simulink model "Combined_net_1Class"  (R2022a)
settings: Solver=FixedStepAuto  StartTime=0.0  StopTime=simtime  FixedStep=1  RelTol=1e-3
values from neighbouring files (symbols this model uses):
  net = closeloop(net)    [Loadnet.m]
  SOH_predict = double(ans.SOHout(simtime))    [SimulationCycle.m]
undefined symbols (not defined in the file or in its folder): dSOC_mu_CC, dSOC_sig_CC, dv_mu_CC, dv_sig_CC, SOC_mu_CC, SOC_sig_CC, SOE_mu_CC, SOE_sig_CC, Step2_Simulink_Models, Thesis
libraries: neural x35, deeplib x1

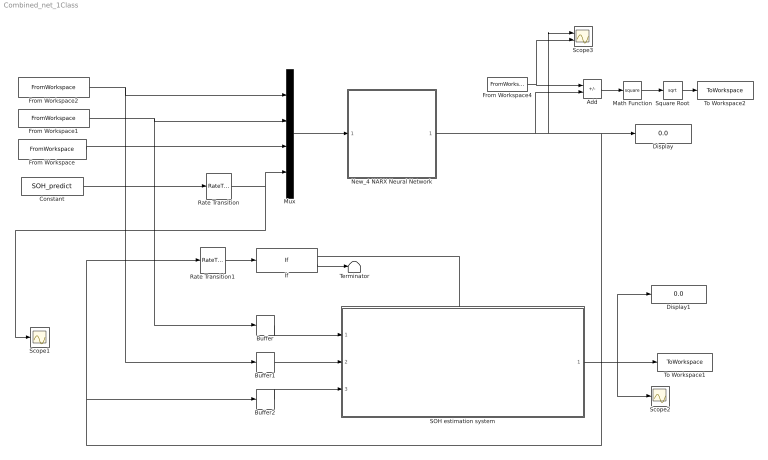
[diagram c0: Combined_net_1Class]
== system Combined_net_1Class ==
  Add : Sum  Inputs=+-
  Buffer : Buffer  N=120  OutputFrames=off
  Buffer1 : Buffer  N=120  OutputFrames=off
  Buffer2 : Buffer  N=120  OutputFrames=off
  Constant : Constant  Value=SOH_predict
  Display : Display
  Display1 : Display
  From Workspace : FromWorkspace  VariableName=Temperature
  From Workspace1 : FromWorkspace  VariableName=Voltage  SampleTime=1
  From Workspace2 : FromWorkspace  VariableName=Current  SampleTime=1
  From Workspace4 : FromWorkspace  VariableName=SOC_GT
  If : If  IfExpression=u1 < 0.6
  Math Function : Math  Operator=square
  Mux : Mux
  New_4 NARX Neural Network : Subsystem  mask{pi_input_1_delayed_1=[0;0;0;0], ai_layer_2_delayed_1=0}
      mask prompts: pi_input_1_delayed_1 "Preprocessed initial input 1 state at timestep 0."; ai_layer_2_delayed_1 "Initial layer 2 state at timestep 0."
      mask help: NARX Neural Network
  Rate Transition : RateTransition  OutPortSampleTime=1
  Rate Transition1 : RateTransition  OutPortSampleTime=1
  SOH estimation system : Subsystem
  Scope1 : Scope
  Scope2 : Scope
  Scope3 : Scope  NumInputPorts=2
  Square Root : Sqrt
  Terminator : Terminator
  To Workspace1 : ToWorkspace  VariableName=SOHout  SampleTime=-1
  To Workspace2 : ToWorkspace  VariableName=SOC_abserror  SampleTime=-1
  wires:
  Mux/1 -> New_4 NARX Neural Network/1(x)
  From Workspace/1 -> Mux/3
  Buffer/1 -> SOH estimation system/1(V)
  From Workspace1/1 -> Mux/2, Buffer/1
  If/1 -> SOH estimation system/Action
  Buffer2/1 -> SOH estimation system/3(SOC)
  Buffer1/1 -> SOH estimation system/2(I)
  Rate Transition1/1 -> If/1
  From Workspace2/1 -> Mux/1, Buffer1/1
  If/2 -> Terminator/1
  Constant/1 -> Rate Transition/1
  SOH estimation system/1(SOH) -> Scope2/1, To Workspace1/1, Display1/1
  Rate Transition/1 -> Mux/4, Scope1/1
  Math Function/1 -> Square Root/1
  Add/1 -> Math Function/1
  New_4 NARX Neural Network/1(y) -> Add/2, Scope3/1, Rate Transition1/1, Buffer2/1, Display/1
  Square Root/1 -> To Workspace2/1
  From Workspace4/1 -> Add/1, Scope3/2

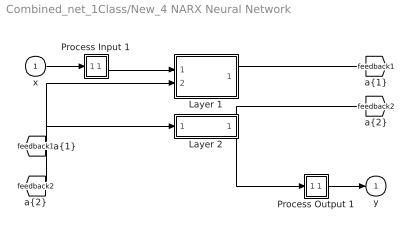
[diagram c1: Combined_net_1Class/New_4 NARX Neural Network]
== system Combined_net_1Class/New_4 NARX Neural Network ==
  x : Inport  PortDimensions=4  SampleTime=1
  Layer 1 : Subsystem
  Layer 2 : Subsystem
  Process Input 1 : Subsystem
  Process Output 1 : Subsystem
  y : Outport  InitialOutput=0
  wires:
  x/1 -> Process Input 1/1(x)
  Process Output 1/1(y) -> y/1
  Process Input 1/1(p) -> Layer 1/1("p{1}")
  Layer 1/1("a{1}") -> [feedback1]
  [feedback1] -> Layer 2/1("a{1} ")
  Layer 2/1("a{2}") -> [feedback2], Process Output 1/1(a)
  [feedback2] -> Layer 1/2("a{2} ")

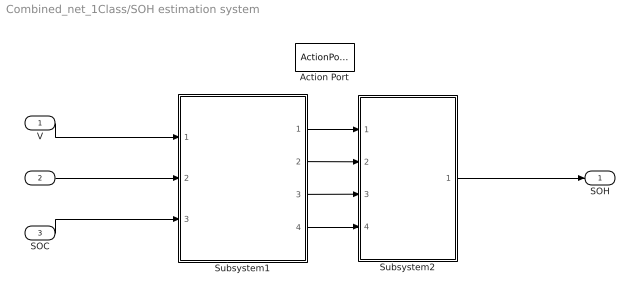
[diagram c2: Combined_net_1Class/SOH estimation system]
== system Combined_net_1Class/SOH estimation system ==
  V : Inport
  I : Inport  Port=2
  SOC : Inport  Port=3
  Action Port : ActionPort  ActionPortLabel=if(u1 < 0.6)
  Subsystem1 : Subsystem
  Subsystem2 : Subsystem
  SOH : Outport
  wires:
  Subsystem1/4(SOE) -> Subsystem2/4(SOE)
  Subsystem1/1(dSOC) -> Subsystem2/1(dSOC)
  Subsystem1/2(dv) -> Subsystem2/2(dv)
  Subsystem1/3(SOC) -> Subsystem2/3(SOC)
  Subsystem2/1(SOH) -> SOH/1
  V/1 -> Subsystem1/1(V_03)
  I/1 -> Subsystem1/2(I_03)
  SOC/1 -> Subsystem1/3(SOC_03)

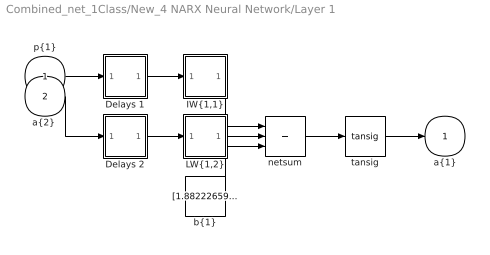
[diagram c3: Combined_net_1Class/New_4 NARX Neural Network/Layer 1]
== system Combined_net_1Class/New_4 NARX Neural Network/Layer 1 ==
  "p{1}" : Inport  PortDimensions=4  SampleTime=1
  "a{2} " : Inport  Port=2  PortDimensions=1  SampleTime=1
  Delays 1 : Subsystem
  Delays 2 : Subsystem
  "IW{1,1}" : Subsystem
  "LW{1,2}" : Subsystem
  "b{1}" : Constant  Value=[1.8822265945278056076261918860836885869503021240234375;-1.6332926436185550844726321884081698954105377197265625;-1.3416753095284523755736927341786213219165802001953125;0.6041072172283656893654324449016712605953216552734375;-0.1437522046735665026684358736019930802285671234130859375;-0.706093682503903696812130874604918062686920166015625;-0.32497208659573073585846714195213280618190765380859375;-0.355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
  netsum : Sum  Inputs=3  InputSameDT=on  SaturateOnIntegerOverflow=on
  tansig : neural/Transfer Functions/tansig
  "a{1}" : Outport  InitialOutput=[0;0;0;0;0;0;0;0;0;0;0;0;0;0;0]
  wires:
  "p{1}"/1 -> Delays 1/1("p{1}")
  Delays 1/1("pd{1,1}") -> "IW{1,1}"/1("pd{1,1}")
  "IW{1,1}"/1("iz{1,1}") -> netsum/1
  "a{2} "/1 -> Delays 2/1("p{1}")
  Delays 2/1("pd{1,2}") -> "LW{1,2}"/1("ad{1,2}")
  "LW{1,2}"/1("lz{1,2}") -> netsum/2
  "b{1}"/1 -> netsum/3
  netsum/1 -> tansig/1
  tansig/1 -> "a{1}"/1

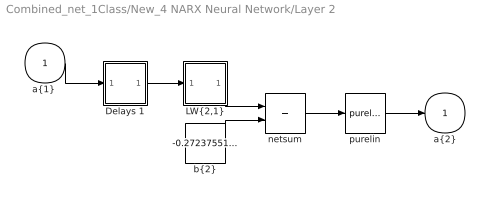
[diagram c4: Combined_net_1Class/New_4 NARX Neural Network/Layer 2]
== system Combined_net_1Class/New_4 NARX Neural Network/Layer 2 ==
  "a{1} " : Inport  PortDimensions=15  SampleTime=1
  Delays 1 : Subsystem
  "LW{2,1}" : Subsystem
  "b{2}" : Constant  Value=-0.272375519140338695489589326825807802379131317138671875
  netsum : Sum  Inputs=2  InputSameDT=on  SaturateOnIntegerOverflow=on
  purelin : neural/Transfer Functions/purelin
  "a{2}" : Outport  InitialOutput=0
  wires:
  "a{1} "/1 -> Delays 1/1("p{2}")
  Delays 1/1("pd{2,1}") -> "LW{2,1}"/1("ad{2,1}")
  "LW{2,1}"/1("lz{2,1}") -> netsum/1
  "b{2}"/1 -> netsum/2
  netsum/1 -> purelin/1
  purelin/1 -> "a{2}"/1

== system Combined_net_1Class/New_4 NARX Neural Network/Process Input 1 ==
  x : Inport  PortDimensions=4  SampleTime=1
  mapminmax : neural/Processing Functions/mapminmax  xmin=[-4.92400000000000037658764995285;2.50570000000000003836930773105;17.1380000000000016768808563938;0.835541218929458540110033482051]  xmax=[1.59400000000000008348877145181;4.1652000000000004575895218295;31.5220000000000020179413695587;1.02410814058582477770187324495]  ymin=-1  ymax=1
  p : Outport  PortDimensions=4  SampleTime=1
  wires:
  x/1 -> mapminmax/1
  mapminmax/1 -> p/1

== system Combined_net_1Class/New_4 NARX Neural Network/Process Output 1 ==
  a : Inport  PortDimensions=1  SampleTime=1
  mapminmax_reverse : neural/Processing Functions/mapminmax_reverse  xmin=-4.21949321457851519659313158095e-06  xmax=1.00000776066564278643511443079  ymin=-1  ymax=1
  y : Outport  PortDimensions=1  SampleTime=1
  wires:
  a/1 -> mapminmax_reverse/1
  mapminmax_reverse/1 -> y/1

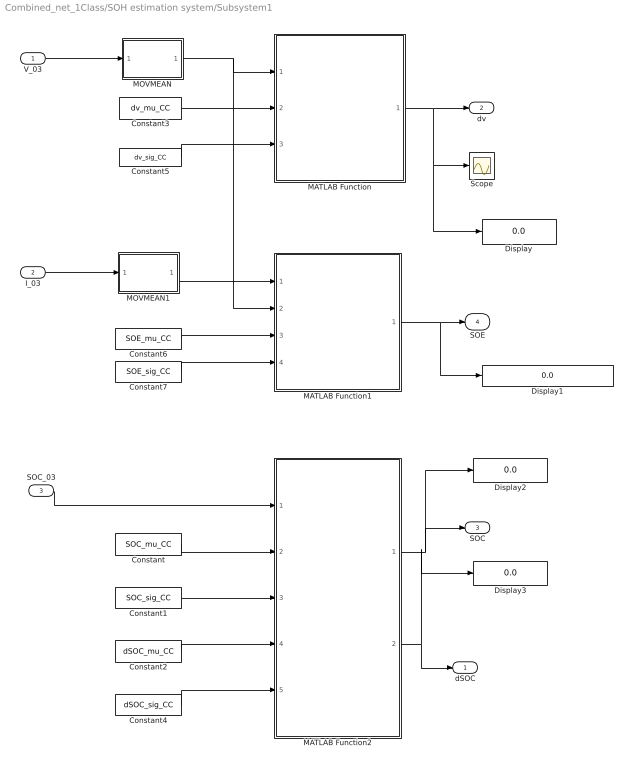
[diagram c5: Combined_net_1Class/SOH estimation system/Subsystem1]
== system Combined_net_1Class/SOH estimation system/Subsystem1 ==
  V_03 : Inport
  I_03 : Inport  Port=2
  SOC_03 : Inport  Port=3
  Constant : Constant  Value=SOC_mu_CC
  Constant1 : Constant  Value=SOC_sig_CC
  Constant2 : Constant  Value=dSOC_mu_CC
  Constant3 : Constant  Value=dv_mu_CC
  Constant4 : Constant  Value=dSOC_sig_CC
  Constant5 : Constant  Value=dv_sig_CC
  Constant6 : Constant  Value=SOE_mu_CC
  Constant7 : Constant  Value=SOE_sig_CC
  Display{,1..3} (4 alike) : Display
  MATLAB Function : MATLAB Function  TreatAsAtomicUnit=on
  MATLAB Function1 : MATLAB Function  TreatAsAtomicUnit=on
  MATLAB Function2 : MATLAB Function  TreatAsAtomicUnit=on
  MOVMEAN : MATLAB Function  TreatAsAtomicUnit=on
  MOVMEAN1 : MATLAB Function  TreatAsAtomicUnit=on
  Scope : Scope
  dSOC : Outport
  dv : Outport  Port=2
  SOC : Outport  Port=3
  SOE : Outport  Port=4
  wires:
  Constant4/1 -> MATLAB Function2/5(dSOC_sig_CC)
  Constant6/1 -> MATLAB Function1/3(SOE_mu_CC)
  Constant7/1 -> MATLAB Function1/4(SOE_sig_CC)
  Constant2/1 -> MATLAB Function2/4(dSOC_mu_CC)
  Constant5/1 -> MATLAB Function/3(dv_sig_CC)
  MATLAB Function2/2(dSOC) -> Display3/1, dSOC/1
  MATLAB Function/1(dV) -> Display/1, Scope/1, dv/1
  MATLAB Function2/1(SOC) -> Display2/1, SOC/1
  Constant3/1 -> MATLAB Function/2(dv_mu_CC)
  V_03/1 -> MOVMEAN/1(V)
  I_03/1 -> MOVMEAN1/1(I)
  Constant1/1 -> MATLAB Function2/3(SOC_sig_CC)
  Constant/1 -> MATLAB Function2/2(SOC_mu_CC)
  MATLAB Function1/1(SOE) -> Display1/1, SOE/1
  MOVMEAN/1(V_filt) -> MATLAB Function/1(V_03), MATLAB Function1/2(V_03)
  MOVMEAN1/1(I_filt) -> MATLAB Function1/1(I_03)
  SOC_03/1 -> MATLAB Function2/1(SOC_03)

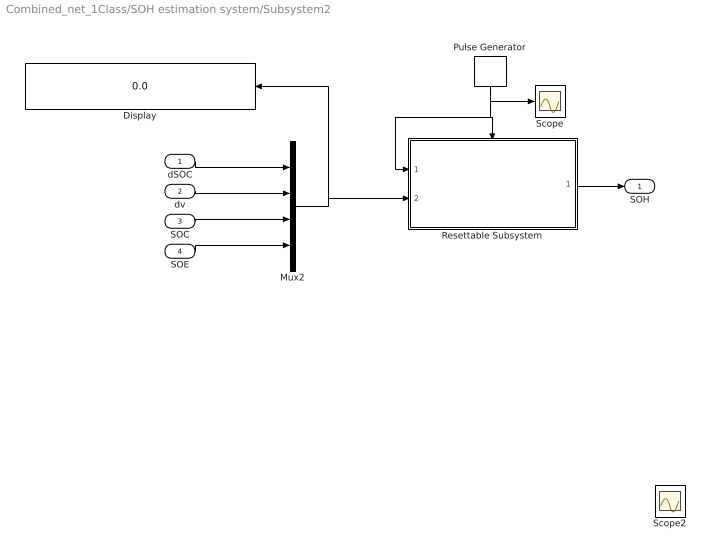
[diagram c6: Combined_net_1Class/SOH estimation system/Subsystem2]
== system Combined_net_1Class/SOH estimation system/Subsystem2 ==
  dSOC : Inport
  dv : Inport  Port=2
  SOC : Inport  Port=3
  SOE : Inport  Port=4
  Display : Display
  Mux2 : Mux
  Pulse Generator : DiscretePulseGenerator  PulseType=Time based  Period=120  PulseWidth=1/120*100  PhaseDelay=119
  Resettable Subsystem : Subsystem  TreatAsAtomicUnit=on
  Scope : Scope
  Scope2 : Scope
  SOH : Outport
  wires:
  Mux2/1 -> Display/1, Resettable Subsystem/2(Input1)
  dSOC/1 -> Mux2/1
  dv/1 -> Mux2/2
  SOC/1 -> Mux2/3
  SOE/1 -> Mux2/4
  Pulse Generator/1 -> Resettable Subsystem/1(Input), Resettable Subsystem/Reset, Scope/1
  Resettable Subsystem/1(Out1) -> SOH/1

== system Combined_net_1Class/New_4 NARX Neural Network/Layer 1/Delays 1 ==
  "p{1}" : Inport  PortDimensions=4  SampleTime=1
  Delay 1 : UnitDelay  InitialCondition=pi_input_1_delayed_1
  mux : Mux  Inputs=2
  "pd{1,1}" : Outport
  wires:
  "p{1}"/1 -> Delay 1/1, mux/1
  Delay 1/1 -> mux/2
  mux/1 -> "pd{1,1}"/1

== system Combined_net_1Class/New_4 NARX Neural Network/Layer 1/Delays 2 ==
  "p{1}" : Inport  PortDimensions=1  SampleTime=1
  Delay 1 : UnitDelay  InitialCondition=ai_layer_2_delayed_1
  mux : Mux  Inputs=1
  "pd{1,2}" : Outport
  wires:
  "p{1}"/1 -> Delay 1/1
  Delay 1/1 -> mux/1
  mux/1 -> "pd{1,2}"/1

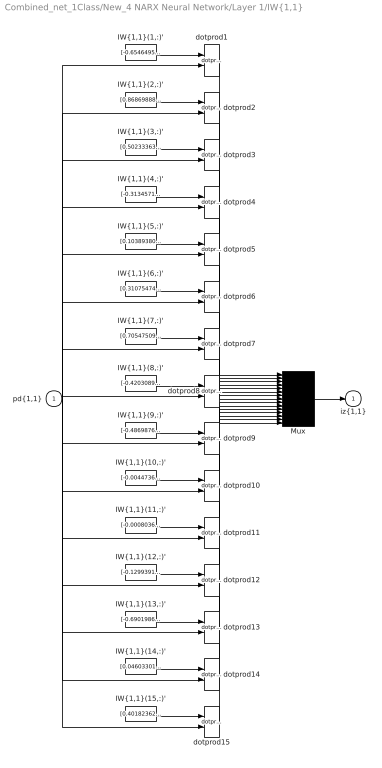
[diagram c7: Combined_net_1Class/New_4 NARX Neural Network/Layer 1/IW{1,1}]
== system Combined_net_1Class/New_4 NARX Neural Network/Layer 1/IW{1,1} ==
  "pd{1,1}" : Inport  PortDimensions=8  SampleTime=1
  "IW{1,1}(1,:)'" : Constant  Value=[-0.65464958479642942901222113505355082452297210693359375;-0.65337619102749877608715678434236906468868255615234375;-0.27677406513585223191142858922830782830715179443359375;0.699544740445478652191013679839670658111572265625;-0.5327508487652377056065233773551881313323974609375;0.655183920476839265489843455725349485874176025390625;0.54512357541839839836228520653094165027141571044921875;0.732399389771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
  "IW{1,1}(10,:)'" : Constant  Value=[-0.004473615007626346833091712795749117503874003887176513671875;0.037970600901949515260103140690262080170214176177978515625;0.000622190521338159062240957819511777415755204856395721435546875;-0.73937293258495884185066415739129297435283660888671875;0.006270143855257244956680207081944899982772767543792724609375;-0.0434914184436572259784270499949343502521514892578125;-0.000978375828634564905297854586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
  "IW{1,1}(11,:)'" : Constant  Value=[-0.000803688640588731575790937267100844110245816409587860107421875;0.007304655688605474032903952519291124190203845500946044921875;0.000179303297634150521529250443819591964711435139179229736328125;-0.64174790841768747373663472899352200329303741455078125;0.00110522572626375425834666099689229668001644313335418701171875;-0.0086662725370479885833585598220452084206044673919677734375;-0.0002161151422075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
  "IW{1,1}(12,:)'" : Constant  Value=[-0.1299391138224756103713986021830351091921329498291015625;-0.3108468188756159378272059257142245769500732421875;-0.301381656439640599476348370444611646234989166259765625;0.813926715557872437756259387242607772350311279296875;0.79444213433619748077063604796421714127063751220703125;-0.74333106820964023331299586061504669487476348876953125;-0.93001715117281469336063537411973811686038970947265625;0.773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
  "IW{1,1}(13,:)'" : Constant  Value=[-0.69019861384391345549005336579284630715847015380859375;0.303517311344015328078427273794659413397312164306640625;-0.11588968500930464655684914987432421185076236724853515625;0.0333233741271399541705733327034977264702320098876953125;0.34215290948315502106424901285208761692047119140625;0.719303753429601844260332654812373220920562744140625;0.1932183998067463492898099275407730601727962493896484375;0.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
  "IW{1,1}(14,:)'" : Constant  Value=[0.046033014342807855590056220762562588788568973541259765625;-0.320009483124574500845227476020227186381816864013671875;-0.0037827151657194740298761903574131792993284761905670166015625;-0.48998833707874134280046973799471743404865264892578125;-0.0559539845377299560613693074628827162086963653564453125;0.35603064580821264240029222492012195289134979248046875;0.004948006288950728380482413371055372408591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
  "IW{1,1}(15,:)'" : Constant  Value=[0.40182362320964504220910384901799261569976806640625;0.443797221498127114625020794846932403743267059326171875;0.404736354887146154712951329202041961252689361572265625;-0.5444547322933590560722905138391070067882537841796875;-0.499221102235928693158228952597710303962230682373046875;0.326541136120923447538899608844076283276081085205078125;-0.78482570856269562309392995302914641797542572021484375;0.36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
  "IW{1,1}(2,:)'" : Constant  Value=[0.86869888871761968829332545283250510692596435546875;0.72024101342312529805411713823559693992137908935546875;0.53978291332661820778326955405646003782749176025390625;1.0762178046281662968652881318121217191219329833984375;-0.5937142553320791105164744294597767293453216552734375;-0.04866153831105286819980193513401900418102741241455078125;0.028861609457539870449149788100839941762387752532958984375;0.6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
  "IW{1,1}(3,:)'" : Constant  Value=[0.502333636054542953530699378461576998233795166015625;-0.04217064256693146828691709515624097548425197601318359375;0.97775496427980745917096783159649930894374847412109375;0.0765530654322205961204161894784192554652690887451171875;-0.9206174201497259179660659356159158051013946533203125;-0.86991362119887083448332987245521508157253265380859375;-0.697857414960799449232808910892345011234283447265625;0.3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
  "IW{1,1}(4,:)'" : Constant  Value=[-0.31345714847786154688691340197692625224590301513671875;0.85034755000740480657128728125826455652713775634765625;0.56028050229703418860793817657395265996456146240234375;-0.037903152207868197332008008970660739578306674957275390625;-0.389621350223876616869489453165442682802677154541015625;-0.558085972171615818382406359887681901454925537109375;0.328888134142325483377788941652397625148296356201171875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
  "IW{1,1}(5,:)'" : Constant  Value=[0.10389380656564677074538138867865200154483318328857421875;-0.71531407808736535702820447113481350243091583251953125;-0.00881952900832292351063212976214344962500035762786865234375;-0.42724834169698355790245614116429351270198822021484375;-0.12428511357538195303273909075869596563279628753662109375;0.78620701918519320106071290865656919777393341064453125;0.012385218222176220051466977167820004979148507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
  "IW{1,1}(6,:)'" : Constant  Value=[0.31075474918349199615619227188290096819400787353515625;-0.86954687162722421600591360402177087962627410888671875;-0.227267153693776868816911473913933150470256805419921875;-0.46922022354537407107244462167727760970592498779296875;0.84939914624888890326559476307011209428310394287109375;-0.34023298555811376520097155662369914352893829345703125;-0.96089900795011995437988616686197929084300994873046875;0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
  "IW{1,1}(7,:)'" : Constant  Value=[0.70547509207102432338132302902522496879100799560546875;0.5333216507004916451251119724474847316741943359375;0.241259959791017164487669788286439143121242523193359375;0.7234565154870693515221091729472391307353973388671875;0.88144459725232271463113420395529828965663909912109375;-0.5530186873877471764870961123961023986339569091796875;-0.49338163591327732770963621078408323228359222412109375;-0.8750598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
  "IW{1,1}(8,:)'" : Constant  Value=[-0.420308996663344147659557847873657010495662689208984375;-1.00456689250621433728838383103720843791961669921875;-0.557251798636304584988465649075806140899658203125;-0.07655558877503908232764473495990387164056301116943359375;-0.77595128658275935862320693559013307094573974609375;0.6684410342356186252033012351603247225284576416015625;-0.16022457961280556215655224150395952165126800537109375;-0.580934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
  "IW{1,1}(9,:)'" : Constant  Value=[-0.486987618942922473319612208797479979693889617919921875;0.96359550467118404437627532388432882726192474365234375;-0.073130027070734737737467412443947978317737579345703125;-1.0254000463140282572993555731954984366893768310546875;-0.049334409015149995048066244862638995982706546783447265625;0.0794147500705200959369989277547574602067470550537109375;-0.2092932986342730117268473577496479265391826629638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
  Mux : Mux  Inputs=15
  dotprod{1..15} (15 alike) : neural/Weight Functions/dotprod
  "iz{1,1}" : Outport
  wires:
  "IW{1,1}(1,:)'"/1 -> dotprod1/1
  "pd{1,1}"/1 -> dotprod1/2, dotprod2/2, dotprod3/2, dotprod4/2, dotprod5/2, dotprod6/2, dotprod7/2, dotprod8/2, dotprod9/2, dotprod10/2, dotprod11/2, dotprod12/2, dotprod13/2, dotprod14/2, dotprod15/2
  dotprod1/1 -> Mux/1
  "IW{1,1}(2,:)'"/1 -> dotprod2/1
  dotprod2/1 -> Mux/2
  "IW{1,1}(3,:)'"/1 -> dotprod3/1
  dotprod3/1 -> Mux/3
  "IW{1,1}(4,:)'"/1 -> dotprod4/1
  dotprod4/1 -> Mux/4
  "IW{1,1}(5,:)'"/1 -> dotprod5/1
  dotprod5/1 -> Mux/5
  "IW{1,1}(6,:)'"/1 -> dotprod6/1
  dotprod6/1 -> Mux/6
  "IW{1,1}(7,:)'"/1 -> dotprod7/1
  dotprod7/1 -> Mux/7
  "IW{1,1}(8,:)'"/1 -> dotprod8/1
  dotprod8/1 -> Mux/8
  "IW{1,1}(9,:)'"/1 -> dotprod9/1
  dotprod9/1 -> Mux/9
  "IW{1,1}(10,:)'"/1 -> dotprod10/1
  dotprod10/1 -> Mux/10
  "IW{1,1}(11,:)'"/1 -> dotprod11/1
  dotprod11/1 -> Mux/11
  "IW{1,1}(12,:)'"/1 -> dotprod12/1
  dotprod12/1 -> Mux/12
  "IW{1,1}(13,:)'"/1 -> dotprod13/1
  dotprod13/1 -> Mux/13
  "IW{1,1}(14,:)'"/1 -> dotprod14/1
  dotprod14/1 -> Mux/14
  "IW{1,1}(15,:)'"/1 -> dotprod15/1
  dotprod15/1 -> Mux/15
  Mux/1 -> "iz{1,1}"/1

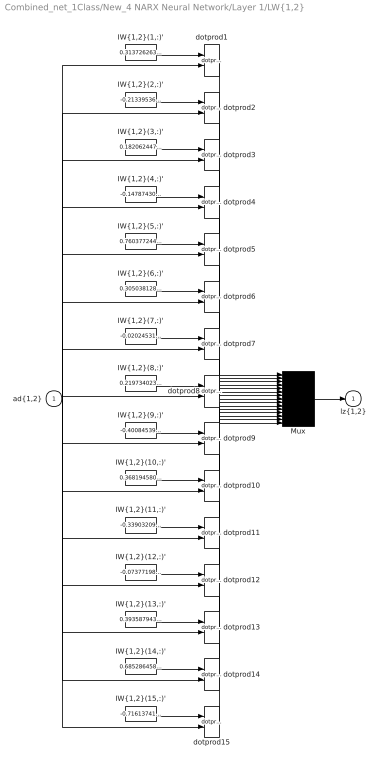
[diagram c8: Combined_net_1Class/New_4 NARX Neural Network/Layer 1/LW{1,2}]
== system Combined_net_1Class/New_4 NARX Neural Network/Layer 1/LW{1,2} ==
  "ad{1,2}" : Inport  PortDimensions=1  SampleTime=1
  "IW{1,2}(1,:)'" : Constant  Value=0.313726263793036863614105413944344036281108856201171875
  "IW{1,2}(10,:)'" : Constant  Value=0.368194580241390401198486870271153748035430908203125
  "IW{1,2}(11,:)'" : Constant  Value=-0.33903209028859737639294280597823671996593475341796875
  "IW{1,2}(12,:)'" : Constant  Value=-0.073771982169325178713137347585870884358882904052734375
  "IW{1,2}(13,:)'" : Constant  Value=0.39358794392944795870192820075317285954952239990234375
  "IW{1,2}(14,:)'" : Constant  Value=0.685286458039714663215136170038022100925445556640625
  "IW{1,2}(15,:)'" : Constant  Value=-0.7161374180503587982826729785301722586154937744140625
  "IW{1,2}(2,:)'" : Constant  Value=-0.213395363259064108074625210065278224647045135498046875
  "IW{1,2}(3,:)'" : Constant  Value=0.1820624470642757675165057662525214254856109619140625
  "IW{1,2}(4,:)'" : Constant  Value=-0.1478743086424599562089809978715493343770503997802734375
  "IW{1,2}(5,:)'" : Constant  Value=0.76037724464155143078158971547964029014110565185546875
  "IW{1,2}(6,:)'" : Constant  Value=0.305038128522850116031150946582783944904804229736328125
  "IW{1,2}(7,:)'" : Constant  Value=-0.02024531678997439076983511085927602834999561309814453125
  "IW{1,2}(8,:)'" : Constant  Value=0.21973402384318896363168960306211374700069427490234375
  "IW{1,2}(9,:)'" : Constant  Value=-0.400845396189503710981938411350711248815059661865234375
  Mux : Mux  Inputs=15
  dotprod{1..15} (15 alike) : neural/Weight Functions/dotprod
  "lz{1,2}" : Outport
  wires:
  "IW{1,2}(1,:)'"/1 -> dotprod1/1
  "ad{1,2}"/1 -> dotprod1/2, dotprod2/2, dotprod3/2, dotprod4/2, dotprod5/2, dotprod6/2, dotprod7/2, dotprod8/2, dotprod9/2, dotprod10/2, dotprod11/2, dotprod12/2, dotprod13/2, dotprod14/2, dotprod15/2
  dotprod1/1 -> Mux/1
  "IW{1,2}(2,:)'"/1 -> dotprod2/1
  dotprod2/1 -> Mux/2
  "IW{1,2}(3,:)'"/1 -> dotprod3/1
  dotprod3/1 -> Mux/3
  "IW{1,2}(4,:)'"/1 -> dotprod4/1
  dotprod4/1 -> Mux/4
  "IW{1,2}(5,:)'"/1 -> dotprod5/1
  dotprod5/1 -> Mux/5
  "IW{1,2}(6,:)'"/1 -> dotprod6/1
  dotprod6/1 -> Mux/6
  "IW{1,2}(7,:)'"/1 -> dotprod7/1
  dotprod7/1 -> Mux/7
  "IW{1,2}(8,:)'"/1 -> dotprod8/1
  dotprod8/1 -> Mux/8
  "IW{1,2}(9,:)'"/1 -> dotprod9/1
  dotprod9/1 -> Mux/9
  "IW{1,2}(10,:)'"/1 -> dotprod10/1
  dotprod10/1 -> Mux/10
  "IW{1,2}(11,:)'"/1 -> dotprod11/1
  dotprod11/1 -> Mux/11
  "IW{1,2}(12,:)'"/1 -> dotprod12/1
  dotprod12/1 -> Mux/12
  "IW{1,2}(13,:)'"/1 -> dotprod13/1
  dotprod13/1 -> Mux/13
  "IW{1,2}(14,:)'"/1 -> dotprod14/1
  dotprod14/1 -> Mux/14
  "IW{1,2}(15,:)'"/1 -> dotprod15/1
  dotprod15/1 -> Mux/15
  Mux/1 -> "lz{1,2}"/1

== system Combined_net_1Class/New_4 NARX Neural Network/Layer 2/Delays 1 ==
  "p{2}" : Inport  PortDimensions=15  SampleTime=1
  mux : Mux  Inputs=1
  "pd{2,1}" : Outport
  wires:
  "p{2}"/1 -> mux/1
  mux/1 -> "pd{2,1}"/1

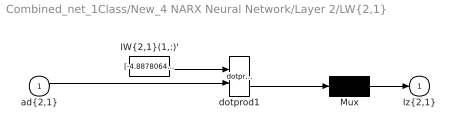
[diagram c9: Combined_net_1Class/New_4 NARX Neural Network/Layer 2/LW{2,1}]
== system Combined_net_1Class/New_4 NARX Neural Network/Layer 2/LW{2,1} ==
  "ad{2,1}" : Inport  PortDimensions=15  SampleTime=1
  "IW{2,1}(1,:)'" : Constant  Value=[-4.887806461353221866572571485676235170103609561920166015625e-05;-3.889267473351513330730166995152785602840594947338104248046875e-05;2.300146907736462680341658904037416277787997387349605560302734375e-05;0.0001665013286308004666382009961722587831900455057621002197265625;0.034971929797273981765926009757095016539096832275390625;7.729981660706192189767664568744720554605009965598583221435546875e-06;6.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
  Mux : Mux  Inputs=1
  dotprod1 : neural/Weight Functions/dotprod
  "lz{2,1}" : Outport
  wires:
  "IW{2,1}(1,:)'"/1 -> dotprod1/1
  "ad{2,1}"/1 -> dotprod1/2
  dotprod1/1 -> Mux/1
  Mux/1 -> "lz{2,1}"/1

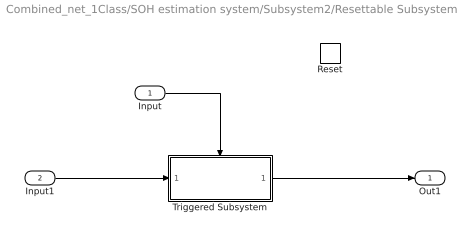
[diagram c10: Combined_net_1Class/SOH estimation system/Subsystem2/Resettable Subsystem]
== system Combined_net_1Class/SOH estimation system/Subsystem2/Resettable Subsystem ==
  Input : Inport
  Input1 : Inport  Port=2
  Reset : ResetPort  DisableCoverage=on
  Triggered Subsystem : Subsystem  TreatAsAtomicUnit=on
  Out1 : Outport
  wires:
  Triggered Subsystem/1(Out1) -> Out1/1
  Input/1 -> Triggered Subsystem/Trigger
  Input1/1 -> Triggered Subsystem/1(u)

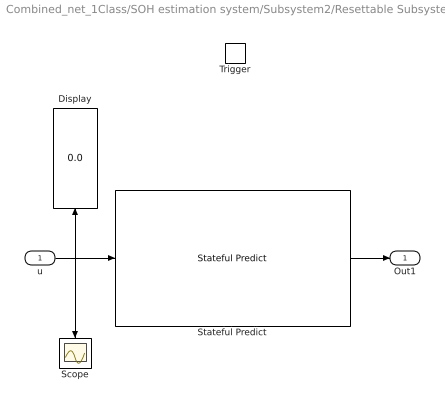
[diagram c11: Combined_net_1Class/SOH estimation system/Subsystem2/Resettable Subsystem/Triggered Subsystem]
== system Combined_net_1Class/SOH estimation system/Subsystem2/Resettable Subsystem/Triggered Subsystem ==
  u : Inport
  Trigger : TriggerPort  TriggerType=falling  VariantControl=(inherit)
  Display : Display
  Scope : Scope
  Stateful Predict : deeplib/Stateful Predict  Network=Network from MAT-file  NetworkFunction=untitled  NetworkFilePath=E:\Thesis\Step2_Simulink_Models\net.mat  InputDataFormats={ '', '' }  SampleTime=-1  ForceInterpretedSim=off  EnableDLNetwork=on
  Out1 : Outport
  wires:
  u/1 -> Stateful Predict/1, Scope/1, Display/1
  Stateful Predict/1 -> Out1/1

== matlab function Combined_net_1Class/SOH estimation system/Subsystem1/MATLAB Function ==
function dV  = V_features(V_03,dv_mu_CC,dv_sig_CC)
dV = ((V_03(120-11)-V_03(1+10))-dv_mu_CC)/dv_sig_CC;
% if dV<-5 || dV>1
%     dV = 0;
% end
end

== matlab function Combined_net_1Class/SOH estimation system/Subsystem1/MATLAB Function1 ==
function SOE  = SOE(I_03,V_03,SOE_mu_CC,SOE_sig_CC)

persistent  E1 E2 E3 E4 dE flag1 flag2 count SOE_reg
if isempty(E1)
    E1 = 0;
    E2 = 0;
    E3 = 0;
    E4 = 0;
    dE = 0;
    flag1 = 0;
    flag2 = 1;
    count = 0;
    SOE_reg = 0;
end

if I_03 ~= 0
    count = count+1;
end

if I_03(1)~=0 && flag1 ==0 && flag2 == 1
    E1 = I_03(1)*V_03(1);
    E2 = I_03(120)*V_03(120);
    flag1 = 1;
    flag2 = 0;
elseif I_03(1)~=0 && flag1 == 1 && flag2 == 0
    E3 = I_03(1)*V_03(1);
    E4 = I_03(120)*V_03(120);
    flag1 = 0;
    flag2 = 1;
end

SOE1 = zeros(1,120);

if count == 1
    SOE1(1) = 0;
elseif mod(count,2) == 1
    dE = (E1-E4)/2;
    SOE1(1) = SOE_reg+dE;
else
    dE = (E3-E2)/2;
    SOE1(1) = SOE_reg+dE;
end

time = linspace(1,120,120);
E = I_03.*V_03;
SOE_cum = cumtrapz(time,E);
k = 2;

for i = 1:119
    SOE1(k) = SOE_cum(i+1)-SOE_cum(i);
    k = k+1;
end

SOE_reg = SOE1(120);

SOE = (SOE1(120-11)-SOE_mu_CC)/SOE_sig_CC;
end

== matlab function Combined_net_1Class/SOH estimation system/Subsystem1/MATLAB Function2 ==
function [SOC,dSOC] = SOC_features(SOC_03,SOC_mu_CC,SOC_sig_CC,dSOC_mu_CC,dSOC_sig_CC)
SOC = (SOC_03(120-11)-SOC_mu_CC)/SOC_sig_CC;
dSOC = ((SOC_03(120-11)-SOC_03(1+10))-dSOC_mu_CC)/dSOC_sig_CC;
if dSOC<-10
    dSOC = 0;
end
end

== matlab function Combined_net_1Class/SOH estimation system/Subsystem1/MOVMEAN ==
function V_filt = filt(V)

V_filt = movmean(V,10);


end

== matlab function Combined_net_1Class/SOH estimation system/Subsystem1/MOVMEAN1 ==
function I_filt = filt(I)

I_filt = movmean(I,10);


end
